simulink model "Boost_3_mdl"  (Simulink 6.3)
settings: Solver=ode45  StartTime=0.0  StopTime=10.0  RelTol=1e-6
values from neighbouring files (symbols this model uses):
  Bg = ones(m,1)    [Boost_3.m]    (also in Boost.m)
  C = 200*microF    (= 0.0002)    [Boost_3.m]    (also in Boost.m)
  Im_0 = In_Con(jj,1)    [Boost_3.m]    (also in Boost.m)
  Lm = eye(m)*L1    [Boost_3.m]    (also in Boost.m)
  R = 100*Ohm    (= 100)    [Boost_3.m]    (also in Boost.m)
  Rm = eye(m)*R1    [Boost_3.m]    (also in Boost.m)
  Tc = 0.00002*sec    (= 2e-05)    [Boost_3.m]    (also in Boost.m = 0.0001)
  Vc_0 = In_Con(jj,2)    [Boost_3.m]    (also in Boost.m)
  Vg = 100*Volt    (= 100)    [Boost_3.m]    (also in Boost.m)
  Vref = 120*Volt    (= 120)    [Boost_3.m]
libraries: simulink x1

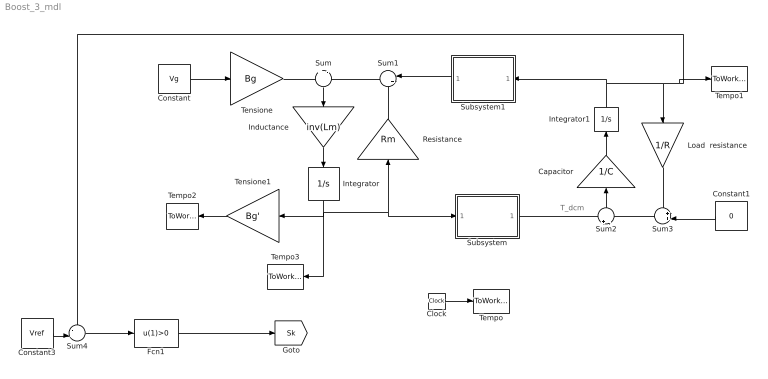
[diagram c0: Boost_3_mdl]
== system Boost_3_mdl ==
  note: T_dcm
  Capacitor : Gain  Orientation=up  Gain=1/C
  Clock : Clock
  Constant : Constant  Value=Vg
  Constant1 : Constant  Orientation=left  Value=0
  Constant3 : Constant  Value=Vref
  Fcn1 : Fcn  Expr=u(1)>0  SampleTime=Tc
  Inductance : Gain  Orientation=down  Gain=inv(Lm)  Multiplication=Matrix(K*u) (u vector)
  Integrator : Integrator  Orientation=down  InitialCondition=Im_0  LimitOutput=on  LowerSaturationLimit=0
  Integrator1 : Integrator  Orientation=up  InitialCondition=Vc_0
  Load  resistance : Gain  Orientation=down  Gain=1/R
  Resistance : Gain  Orientation=up  Gain=Rm  Multiplication=Matrix(K*u) (u vector)
  Subsystem : Subsystem
  Subsystem1 : Subsystem  Orientation=left
  Sum : Sum  Orientation=down  Inputs=+|-
  Sum1 : Sum  Orientation=left  Inputs=|++
  Sum2 : Sum  Orientation=up  Inputs=+|-
  Sum3 : Sum  Orientation=left  Inputs=++|
  Sum4 : Sum  Inputs=-+|
  Tempo : ToWorkspace  VariableName=t  SampleTime=Tc  SaveFormat=Array
  Tempo1 : ToWorkspace  VariableName=Vc  SampleTime=Tc  SaveFormat=Array
  Tempo2 : ToWorkspace  VariableName=Idc  SampleTime=Tc  SaveFormat=Array
  Tempo3 : ToWorkspace  VariableName=Im  SampleTime=Tc  SaveFormat=Array
  Tensione : Gain  Gain=Bg  Multiplication=Matrix(K*u) (u vector)
  Tensione1 : Gain  Orientation=left  Gain=Bg'  Multiplication=Matrix(K*u) (u vector)
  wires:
  Clock/1 -> Tempo/1
  Sum/1 -> Inductance/1
  Inductance/1 -> Integrator/1
  Integrator/1 -> Resistance/1, Subsystem/1(In1), Tempo3/1, Tensione1/1
  Sum1/1 -> Sum/2
  Resistance/1 -> Sum1/2
  Subsystem/1(Out1) -> Sum2/1
  Sum2/1 -> Capacitor/1
  Capacitor/1 -> Integrator1/1
  Integrator1/1 -> Load  resistance/1, Tempo1/1, Sum4/1, Subsystem1/1(In1)
  Load  resistance/1 -> Sum3/1
  Sum3/1 -> Sum2/2
  Constant1/1 -> Sum3/2
  Subsystem1/1(Out1) -> Sum1/1
  Tensione/1 -> Sum/1
  Tensione1/1 -> Tempo2/1
  Constant3/1 -> Sum4/2
  Sum4/1 -> Fcn1/1
  Constant/1 -> Tensione/1
  Fcn1/1 -> [Sk]

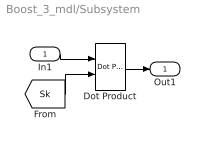
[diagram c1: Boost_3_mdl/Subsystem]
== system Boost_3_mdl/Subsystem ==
  In1 : Inport
  Dot Product : simulink/Math Operations/Dot Product  InputSameDT=on  OutDataType=sfix(16)  OutScaling=2^-10  DoSatur=off
  Out1 : Outport
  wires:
  [Sk] -> Dot Product/2
  In1/1 -> Dot Product/1
  Dot Product/1 -> Out1/1

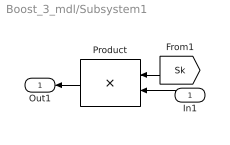
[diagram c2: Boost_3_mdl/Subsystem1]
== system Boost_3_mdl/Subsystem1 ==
  In1 : Inport  Orientation=left
  Product : Product  Orientation=left  Multiplication=Matrix(*)
  Out1 : Outport  Orientation=left
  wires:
  [Sk] -> Product/1
  In1/1 -> Product/2
  Product/1 -> Out1/1
